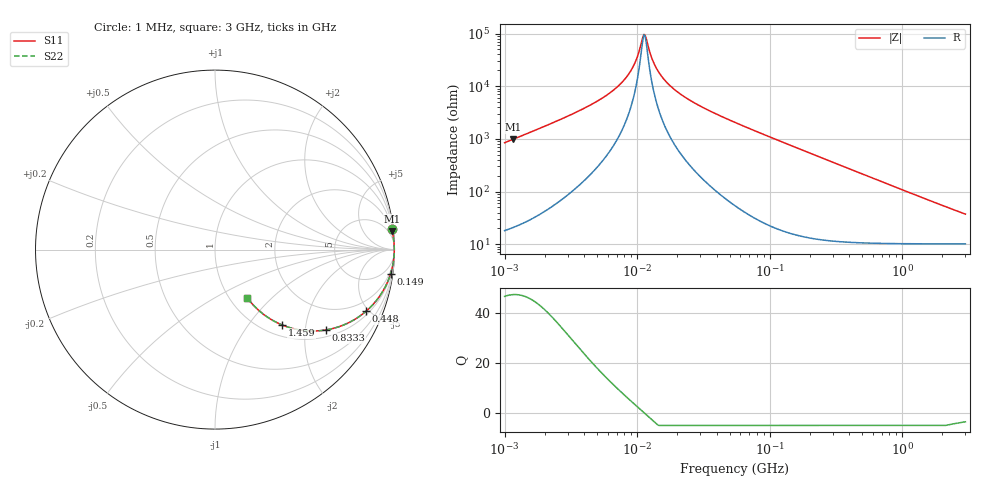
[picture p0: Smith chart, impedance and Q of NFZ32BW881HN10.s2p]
! NFZ32BW881HN10
# Hz S RI R 50
!Freq.(Hz) S11(Real) S11(Imag) S21(Real) S21(Imag) S12(Real) S12(Imag) S22(Real) S22(Imag)
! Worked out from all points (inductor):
!   401 points, 1 MHz to 3 GHz, reference 50 ohm
!   read as one part in series: L = 133 uH near 1.041 MHz
!   highest Q = 47.3 at 1.15 MHz (marker M1), where L = 135 uH
!   self-resonance near 11.27 MHz
!   S11 on the Smith chart (normalised r, x): 1 MHz: 1, +17; 149 MHz: 1, -15; 448 MHz: 1.21, -4.81; 833.3 MHz: 1.21, -2.58; 1.459 GHz: 1.20, -1.48; 3 GHz: 1.20, -0.72
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1000000  0.9838 0.1161  0.0162 -0.1161  0.0162 -0.1161  0.9838 0.1161
1150402  0.9875 0.1011  0.0125 -0.1011  0.0125 -0.1011  0.9875 0.1011
3823119  0.9981 0.0276  0.00188 -0.0276  0.00188 -0.0276  0.9981 0.0276
5938264  0.9987 0.0145  0.00127 -0.0145  0.00127 -0.0145  0.9987 0.0145
8017732  0.9989 0.00742  0.0011 -0.00742  0.0011 -0.00742  0.9989 0.00742
9410094  0.9989 0.00393  0.00105 -0.00393  0.00105 -0.00393  0.9989 0.00393
9992459  0.999 0.00265  0.00104 -0.00265  0.00104 -0.00265  0.999 0.00265
1.082539e7  0.999 0.000966  0.00104 -0.000966  0.00104 -0.000966  0.999 0.000966
1.126754e7  0.999 0.000124  0.00103 -0.000124  0.00103 -0.000124  0.999 0.000124
1.172775e7  0.999 -0.000717  0.00103 0.000717  0.00103 0.000717  0.999 -0.000717
1.29622e7  0.999 -0.00283  0.00104 0.00283  0.00104 0.00283  0.999 -0.00283
1.461624e7  0.9989 -0.0054  0.00107 0.0054  0.00107 0.0054  0.9989 -0.0054
1.750132e7  0.9989 -0.00942  0.00113 0.00942  0.00113 0.00942  0.9989 -0.00942
2.270269e7  0.9987 -0.0158  0.00131 0.0158  0.00131 0.0158  0.9987 -0.0158
5.477226e7  0.9964 -0.0485  0.00363 0.0485  0.00363 0.0485  0.9964 -0.0485
1.49005e8  0.9786 -0.1342  0.0214 0.1342  0.0214 0.1342  0.9786 -0.1342
2.094008e8  0.9595 -0.1851  0.0405 0.1851  0.0405 0.1851  0.9595 -0.1851
4.480278e8  0.842 -0.3432  0.158 0.3432  0.158 0.3432  0.842 -0.3432
8.005644e8  0.6354 -0.4445  0.3646 0.4445  0.3646 0.4445  0.6354 -0.4445
8.332625e8  0.6178 -0.4477  0.3822 0.4477  0.3822 0.4477  0.6178 -0.4477
1.45942e9  0.3732 -0.4196  0.6268 0.4196  0.6268 0.4196  0.3732 -0.4196
3e9  0.1791 -0.2674  0.8209 0.2674  0.8209 0.2674  0.1791 -0.2674
